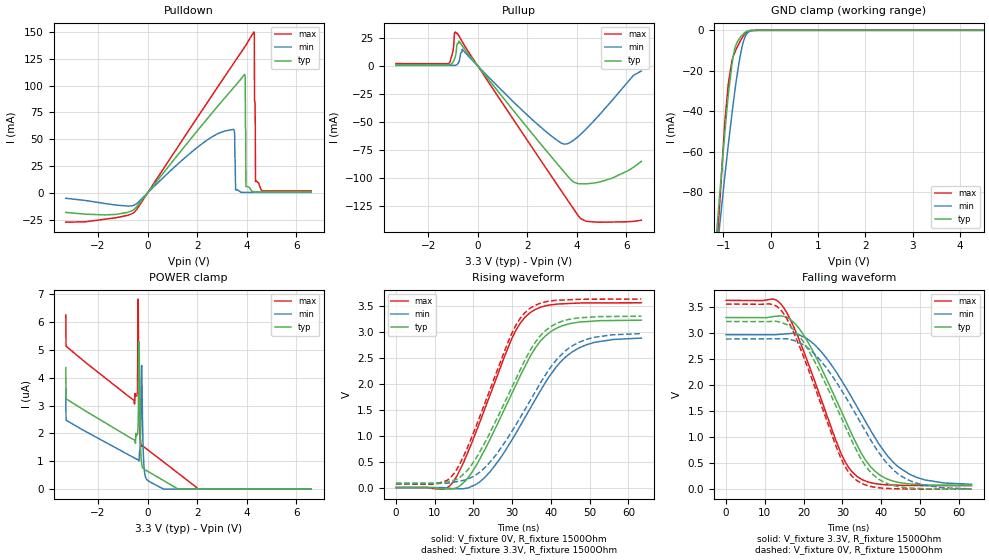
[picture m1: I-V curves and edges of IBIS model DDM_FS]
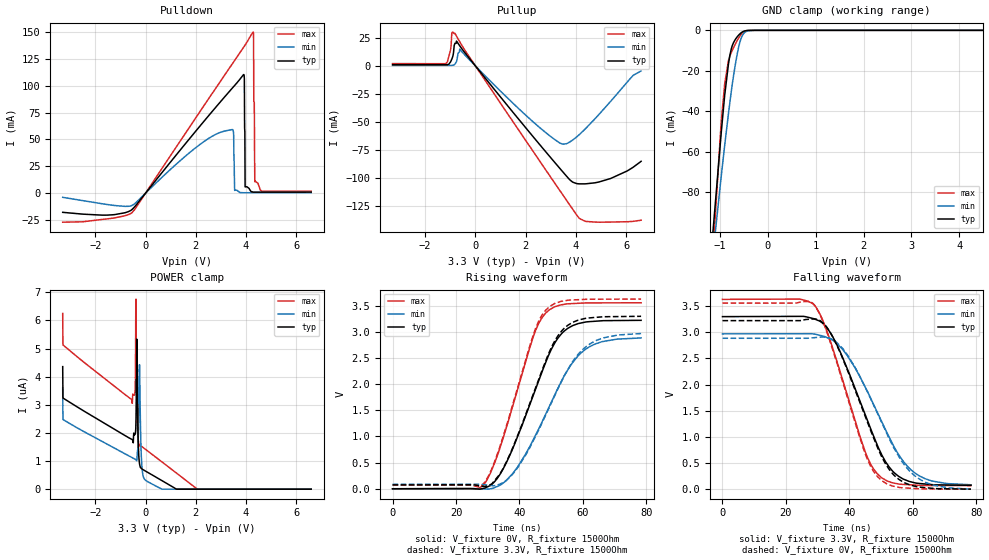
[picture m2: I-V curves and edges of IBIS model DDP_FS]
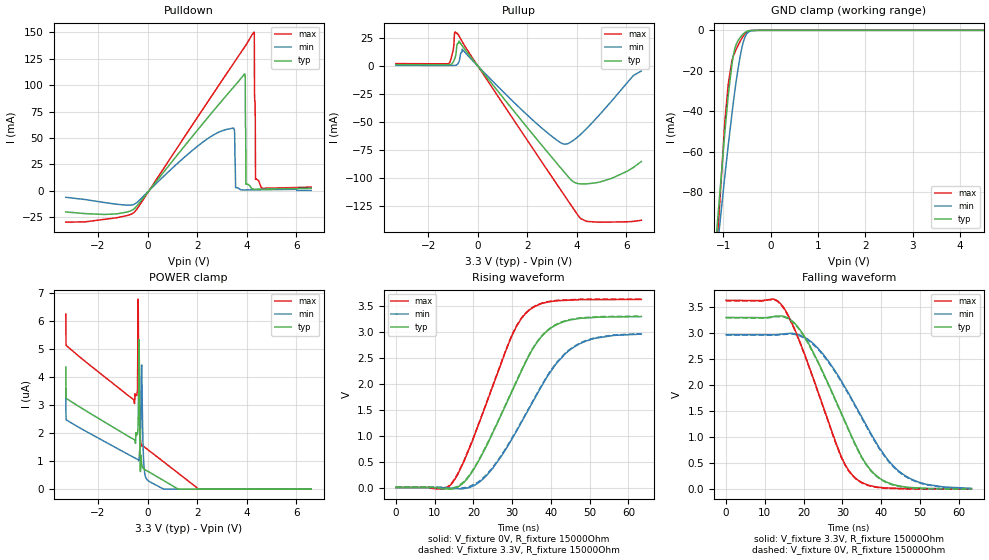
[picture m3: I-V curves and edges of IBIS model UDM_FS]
|Texas Instruments Incorporated
| ISOUSB111 Full/Low Speed Isolated USB Repeater
| Marketing Part # : ISOUSB111
| Package-type: SOIC
| #pins/pkg drawing : 16-pin DW
[IBIS Ver] 4.1
[File name] isousb211.ibs
[File Rev] 1.0
[Date] 09/25/2022
[Source]
| Texas Instruments Incorporated.
| 12500 TI Blvd
| Dallas, TX -75243
[Notes] Revision History:
| Rev 1.0: 09/25/2022
| - Initial version of the model
| - Model generated from simulations in TISPICE/SPECTRE
| - C_comp although listed in numerical order of value are
| obtained from varying PVT conditions. For PVT conditions for
| each specific value refer the buffer description under
| respective [Model]. IBIS model user is responsible for using
| appropriate C_comp to simulate for Signal Integrity.
| - Warnings regarding combined Non-monotonicity of various models have been
| reviewed and considered minor and can be ignored.
[Disclaimer]
| This model is designed as an aid for customers of Texas Instruments.
| TI and its licensors and suppliers make no warranties, either expressed
| or implied, with respect to this model, including the warranties of
| merchantability or fitness for a particular purpose. The model is
| provided solely on an "as is" basis. The entire risk as to its quality
| and performance is with the customer.
| This model is subject to change without notice. Texas Instruments
| Incorporated is not responsible for updating this model.
[Copyright]
(C) Copyright 2022 Texas Instruments Incorporated. All rights reserved.
[Component] ISOUSB211
[Manufacturer] Texas Instruments Incorporated
[Package]
R_pkg 0.05 0.04 0.06
L_pkg 1.5nH 1.2nH 2nH
C_pkg 0.2pF 0.16pF 0.24pF
| pin number (pin name) mapping to model name
[Pin] signal_name  model_name   R_pin   L_pin   C_pin
1 Vbus1 Power 0 0 0
2 V3p3V1 Power 0 0 0
3 GND1 GND 0 0 0
4 V1p8V1 Power 0 0 0
5 Vcc1 Power 0 0 0
6 V2OK NC 0 0 0
7 UDM UDM 0 0 0
8 UDP UDP 0 0 0
9 EQ10 NC 0 0 0
10 EQ11 NC 0 0 0
11 V1p8V1_2 Power 0 0 0
12 GND1 GND 0 0 0
13 CDPENZ1 NC 0 0 0
14 SDA1 NC 0 0 0
15 SDA2 NC 0 0 0
16 CDPENZ2 NC 0 0 0
17 GND2 GND 0 0 0
18 V1p8V2_2 Power 0 0 0
19 EQ21 NC 0 0 0
20 EQ20 NC 0 0 0
21 DDP DDP 0 0 0
22 DDM DDM 0 0 0
23 V1OK NC 0 0 0
24 Vcc2 Power 0 0 0
25 V1p8V2 Power 0 0 0
26 GND2 GND 0 0 0
27 V3p3V2 Power 0 0 0
28 Vbus2 Power 0 0 0
[Model Selector]   UDP
UDP_FS   upstream_positive_full_speed_mode
UDP_LS   upstream_positive_low_speed_mode
DP_EQ0   high_speed_eq0
DP_EQ1   high_speed_eq1
DP_EQ2   high_speed_eq2
DP_EQ3   high_speed_eq3
DP_EQ4   high_speed_eq4
DP_EQ5   high_speed_eq5
DP_EQ6   high_speed_eq6
DP_EQ7   high_speed_eq7
[Model Selector]   UDM
UDM_FS   upstream_negative_full_speed_mode
UDM_LS   upstream_negative_low_speed_mode
DM_EQ0   high_speed_eq0
DM_EQ1   high_speed_eq1
DM_EQ2   high_speed_eq2
DM_EQ3   high_speed_eq3
DM_EQ4   high_speed_eq4
DM_EQ5   high_speed_eq5
DM_EQ6   high_speed_eq6
DM_EQ7   high_speed_eq7
[Model Selector]   DDP
DDP_FS   downstream_positive_full_speed_mode
DDP_LS   downstream_positive_low_speed_mode
DP_EQ0   high_speed_eq0
DP_EQ1   high_speed_eq1
DP_EQ2   high_speed_eq2
DP_EQ3   high_speed_eq3
DP_EQ4   high_speed_eq4
DP_EQ5   high_speed_eq5
DP_EQ6   high_speed_eq6
DP_EQ7   high_speed_eq7
[Model Selector]   DDM
DDM_FS   downstream_negative_full_speed_mode
DDM_LS   downstream_negative_low_speed_mode
DM_EQ0   high_speed_eq0
DM_EQ1   high_speed_eq1
DM_EQ2   high_speed_eq2
DM_EQ3   high_speed_eq3
DM_EQ4   high_speed_eq4
DM_EQ5   high_speed_eq5
DM_EQ6   high_speed_eq6
DM_EQ7   high_speed_eq7
| Models and submodels in the file (24): UDP_LS (I/O), DDM_FS (I/O), DDM_LS (I/O), DDP_FS (I/O), DDP_LS (I/O), UDM_FS (I/O), UDM_LS (I/O), UDP_FS (I/O), DM_EQ0 (Output), DM_EQ1 (Output), DM_EQ2 (Output), DM_EQ3 (Output), DM_EQ4 (Output), DM_EQ5 (Output), DM_EQ6 (Output), DM_EQ7 (Output), DP_EQ0 (Output), DP_EQ1 (Output), DP_EQ2 (Output), DP_EQ3 (Output), DP_EQ4 (Output), DP_EQ5 (Output), DP_EQ6 (Output), DP_EQ7 (Output)
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[Model]   DDM_FS
Model_type   I/O
Polarity   Non-Inverting
Enable   Active-Low
Vinl = 0.8
Vinh = 2
Vmeas = 1.65
Vref = 1.65
Cref = 7pF
Rref = 15000
|   typ   min   max
C_comp   8pF   5pF   10pF
[Voltage Range]   3.3   2.97   3.63
[Temperature Range]   27   150   -40
[Pullup Reference]   3.3   2.97   3.63
[Pulldown Reference]   0   0   -0
[Power Clamp Reference]   3.3   2.97   3.63
[GND Clamp Reference]   0   0   0
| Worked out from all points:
|   slope of the pulldown table from 0 to 0.495 V, typ, clamps not added: 34.2 ohm
|   slope of the pullup table from 0 to 0.495 V, typ, clamps not added: 35.8 ohm
|   GND clamp passes 1 mA (typ) near -0.54 V on its own axis
|   falling waveform, V_fixture 3.3V, R_fixture 1500Ohm: 20-80 % time 12.3ns typ, 14.3ns min, 10.5ns max; typ from 3.3 V to 0.074 V
|   rising waveform, V_fixture 0V, R_fixture 1500Ohm: 20-80 % time 12.7ns typ, 14.1ns min, 11.1ns max; typ from 0 V to 3.22 V
|   rising waveform, V_fixture 3.3V, R_fixture 1500Ohm: 20-80 % time 12.9ns typ, 14.5ns min, 11.1ns max; typ from 0.073 V to 3.3 V
|   falling waveform, V_fixture 0V, R_fixture 1500Ohm: 20-80 % time 12.4ns typ, 14.5ns min, 10.6ns max; typ from 3.22 V to 0 V
[Pulldown]
|   Voltage   I(typ)   I(min)   I(max)
-3.3V     -18.2mA    -5.025mA   -27.3mA
-537.9mV  -15.2mA    -11.4mA    -18.05mA
3.452V    97.57mA    59.15mA    120.1mA
3.551V    100.2mA    2.565mA    123.5mA
3.917V    110.3mA    416.6uA    136mA
3.937V    106.9mA    416.6uA    136.7mA
3.967V    5.849mA    416.6uA    137.7mA
4.283V    1.079mA    416.7uA    149.8mA
4.303V    992.1uA    416.7uA    149.2mA
4.313V    991.4uA    416.7uA    86.59mA
4.353V    991.8uA    416.8uA    10.6mA
6.6V      1.045mA    452.9uA    1.865mA
[GND Clamp]
|   Voltage   I(typ)   I(min)   I(max)
-3.3V     -1.286A    -1.12A     -1.579A
-1.3V     -145.3mA   -147.2mA   -170.6mA
-973.5mV  -52.59mA   -73.66mA   -47.69mA
-894.3mV  -32.06mA   -56.82mA   -26.49mA
-815.1mV  -16.5mA    -41.06mA   -14.88mA
-785.4mV  -12.23mA   -35.46mA   -12.65mA
-735.9mV  -7.575mA   -26.62mA   -9.854mA
-627mV    -3.033mA   -10.97mA   -4.745mA
-567.6mV  -1.539mA   -5.066mA   -2.489mA
-498.3mV  -471.8uA   -1.572mA   -746.7uA
-260.7mV  0A         -5.306uA   0A
6.6V      0A         0A         0A
[Pullup]
|   Voltage   I(typ)   I(min)   I(max)
-3.3V     1.143mA    463.1uA    2.098mA
-1.181V   1.062mA    442.4uA    1.969mA
-993.3mV  3.464mA    442uA      14.04mA
-933.9mV  6.443mA    534.3uA    29.81mA
-815.1mV  20.24mA    1.625mA    29.16mA
-627mV    18.1mA     15mA       21.74mA
1.957V    -54.06mA   -43.1mA    -65.17mA
3.491V    -95.06mA   -70.03mA   -115.7mA
3.868V    -103.9mA   -66.45mA   -128mA
4.382V    -105.5mA   -56.25mA   -139.1mA
5.402V    -100.6mA   -31.33mA   -139.7mA
6.6V      -85.42mA   -4.486mA   -138.1mA
[POWER Clamp]
|   Voltage   I(typ)   I(min)   I(max)
-3.3V     4.356uA    3.599uA    6.245uA
-3.29V    3.24uA     2.477uA    5.129uA
-528mV    1.759uA    1.119uA    3.056uA
-409.2mV  1.967uA    1.064uA    3.479uA
-379.5mV  2.466uA    1.044uA    6.817uA
-349.8mV  5.299uA    1.01uA     3.356uA
-290.4mV  1.653uA    1.775uA    1.768uA
-250.8mV  990.4nA    4.213uA    1.556uA
-171.6mV  742.1nA    1.255uA    1.531uA
-62.7mV   674.2nA    386.2nA    1.457uA
2.056V    0A         0A         4.44nA
6.6V      0A         0A         0A
[Ramp]
R_load = 1500
|   typ   min   max
dV/dt_r   1.93262/1.26758e-08   1.7258/1.41041e-08   2.1342/1.10067e-08
dV/dt_f   1.93485/1.22744e-08   1.7255/1.42298e-08   2.13627/1.05125e-08
[Falling Waveform]
V_fixture = 3.3V
V_fixture_min = 2.97V
V_fixture_max = 3.63V
R_fixture = 1500Ohm
C_fixture = 0F
|   Time   V(typ)   V(min)   V(max)
0s        3.298V     2.969V     3.628V
14.55ns   3.324V     2.979V     3.522V
17.92ns   3.171V     2.984V     3.041V
22.88ns   2.584V     2.773V     2.078V
29.72ns   1.502V     2.098V     678.8mV
33.83ns   844.9mV    1.58V      243.3mV
38.29ns   354.9mV    1.008V     109.5mV
44.81ns   126.3mV    407.8mV    74.94mV
51.52ns   83.59mV    174.8mV    69.48mV
63.33ns   73.73mV    92.92mV    67.43mV
[Rising Waveform]
V_fixture = 0V
V_fixture_min = 0V
V_fixture_max = 0V
R_fixture = 1500Ohm
C_fixture = 0F
|   Time   V(typ)   V(min)   V(max)
0s        7.21nV     276nV      6.379nV
12.02ns   -25.13mV   -1.021mV   -31.53mV
14.55ns   -28.04mV   -21.32mV   87.57mV
17.92ns   127.4mV    -16.65mV   565.1mV
22.88ns   720.2mV    189.9mV    1.502V
30.16ns   1.847V     944.2mV    2.908V
34.59ns   2.517V     1.515V     3.364V
40.02ns   3.004V     2.182V     3.516V
45.64ns   3.165V     2.617V     3.546V
63.33ns   3.221V     2.876V     3.557V
[Rising Waveform]
V_fixture = 3.3V
V_fixture_min = 2.97V
V_fixture_max = 3.63V
R_fixture = 1500Ohm
C_fixture = 0F
|   Time   V(typ)   V(min)   V(max)
0s        73.38mV    83.93mV    67.42mV
10.05ns   74.06mV    82.64mV    70.96mV
15.13ns   142mV      106mV      283.6mV
18.84ns   367mV      174.1mV    839.2mV
24.36ns   1.069V     494.6mV    1.901V
30.07ns   1.952V     1.101V     2.994V
34.4ns    2.607V     1.643V     3.439V
39.75ns   3.089V     2.299V     3.589V
45.64ns   3.249V     2.733V     3.618V
63.33ns   3.298V     2.963V     3.628V
[Falling Waveform]
|Gnd
V_fixture = 0V
V_fixture_min = 0V
V_fixture_max = 0V
R_fixture = 1500Ohm
C_fixture = 0F
|   Time   V(typ)   V(min)   V(max)
0s        3.222V     2.885V     3.557V
11.28ns   3.221V     2.889V     3.561V
14.55ns   3.195V     2.89V      3.404V
18.84ns   2.946V     2.817V     2.761V
22.88ns   2.449V     2.595V     1.969V
29.64ns   1.389V     1.918V     592.2mV
33.63ns   753.5mV    1.42V      172.6mV
39.25ns   198.2mV    720mV      28.06mV
45.64ns   36.48mV    232.3mV    4.575mV
63.33ns   223.6uV    5.519mV    8.818uV
[Model]   DDP_FS
Model_type   I/O
Polarity   Non-Inverting
Enable   Active-Low
Vinl = 0.8
Vinh = 2
Vmeas = 1.65
Vref = 1.65
Cref = 7pF
Rref = 15000
|   typ   min   max
C_comp   8pF   5pF   10pF
[Voltage Range]   3.3   2.97   3.63
[Temperature Range]   27   150   -40
[Pullup Reference]   3.3   2.97   3.63
[Pulldown Reference]   -0   0   0
[Power Clamp Reference]   3.3   2.97   3.63
[GND Clamp Reference]   0   0   0
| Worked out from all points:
|   slope of the pulldown table from 0 to 0.495 V, typ, clamps not added: 34.2 ohm
|   slope of the pullup table from 0 to 0.495 V, typ, clamps not added: 35.8 ohm
|   GND clamp passes 1 mA (typ) near -0.54 V on its own axis
|   falling waveform, V_fixture 3.3V, R_fixture 1500Ohm: 20-80 % time 12.8ns typ, 14.5ns min, 11.1ns max; typ from 3.3 V to 0.073 V
|   rising waveform, V_fixture 0V, R_fixture 1500Ohm: 20-80 % time 12.4ns typ, 14.5ns min, 10.6ns max; typ from 0 V to 3.22 V
|   rising waveform, V_fixture 3.3V, R_fixture 1500Ohm: 20-80 % time 12.3ns typ, 14.2ns min, 10.5ns max; typ from 0.073 V to 3.3 V
|   falling waveform, V_fixture 0V, R_fixture 1500Ohm: 20-80 % time 12.7ns typ, 14.1ns min, 11ns max; typ from 3.22 V to 0 V
[Pulldown]
|   Voltage   I(typ)   I(min)   I(max)
-3.3V     -17.81mA   -3.85mA    -26.98mA
-537.9mV  -15.2mA    -11.4mA    -18.05mA
3.452V    97.57mA    59.13mA    120.1mA
3.551V    100.2mA    2.568mA    123.5mA
3.907V    110.2mA    416.5uA    135.6mA
3.937V    106.3mA    416.5uA    136.7mA
3.967V    5.859mA    416.5uA    137.7mA
4.283V    1.074mA    416.6uA    149.8mA
4.303V    991.3uA    416.6uA    149mA
4.313V    991.1uA    416.6uA    85.12mA
4.353V    991.5uA    416.7uA    10.62mA
6.6V      1.044mA    452.8uA    1.864mA
[GND Clamp]
|   Voltage   I(typ)   I(min)   I(max)
-3.3V     -1.286A    -1.121A    -1.579A
-1.3V     -145.3mA   -147.2mA   -170.6mA
-973.5mV  -52.59mA   -73.66mA   -47.68mA
-894.3mV  -32.06mA   -56.81mA   -26.49mA
-815.1mV  -16.5mA    -41.06mA   -14.88mA
-785.4mV  -12.23mA   -35.46mA   -12.65mA
-735.9mV  -7.575mA   -26.62mA   -9.853mA
-627mV    -3.033mA   -10.97mA   -4.745mA
-567.6mV  -1.539mA   -5.066mA   -2.489mA
-498.3mV  -471.8uA   -1.571mA   -746.6uA
-260.7mV  0A         -5.306uA   0A
6.6V      0A         0A         0A
[Pullup]
|   Voltage   I(typ)   I(min)   I(max)
-3.3V     1.143mA    463.2uA    2.099mA
-1.181V   1.062mA    442.5uA    1.996mA
-993.3mV  3.496mA    442.2uA    14.19mA
-933.9mV  6.482mA    535.1uA    29.92mA
-815.1mV  20.26mA    1.636mA    29.12mA
-627mV    18.09mA    14.99mA    21.7mA
1.957V    -54.04mA   -43.09mA   -65.14mA
3.491V    -95.04mA   -70.01mA   -115.7mA
3.868V    -103.9mA   -66.43mA   -128mA
4.382V    -105.5mA   -56.22mA   -139.1mA
5.392V    -100.7mA   -31.56mA   -139.7mA
6.6V      -85.38mA   -4.479mA   -138.1mA
[POWER Clamp]
|   Voltage   I(typ)   I(min)   I(max)
-3.3V     4.356uA    3.599uA    6.245uA
-3.29V    3.24uA     2.478uA    5.13uA
-528mV    1.759uA    1.119uA    3.053uA
-409.2mV  1.963uA    1.064uA    3.57uA
-379.5mV  2.509uA    1.044uA    6.758uA
-349.8mV  5.335uA    1.011uA    3.278uA
-300.3mV  1.978uA    1.538uA    1.841uA
-250.8mV  984.9nA    4.227uA    1.559uA
-171.6mV  741.8nA    1.249uA    1.531uA
-62.7mV   674.2nA    385.9nA    1.457uA
2.056V    0A         0A         4.445nA
6.6V      0A         0A         0A
[Ramp]
R_load = 1500
|   typ   min   max
dV/dt_r   1.93339/1.2374e-08   1.73122/1.44206e-08   2.13488/1.05473e-08
dV/dt_f   1.93542/1.282e-08   1.73113/1.44351e-08   2.13691/1.10541e-08
[Falling Waveform]
V_fixture = 3.3V
V_fixture_min = 2.97V
V_fixture_max = 3.63V
R_fixture = 1500Ohm
C_fixture = 0F
|   Time   V(typ)   V(min)   V(max)
0s        3.299V     2.969V     3.629V
28.18ns   3.269V     2.972V     3.559V
31.52ns   3.176V     2.93V      3.243V
35.96ns   2.774V     2.79V      2.466V
44.98ns   1.428V     1.953V     717.8mV
48.64ns   866.3mV    1.491V     304.5mV
53.85ns   331.6mV    836.3mV    118.6mV
60.64ns   121mV      310mV      78.34mV
66.13ns   86.39mV    154.8mV    70.52mV
78.33ns   73.35mV    83.9mV     67.4mV
[Rising Waveform]
V_fixture = 0V
V_fixture_min = 0V
V_fixture_max = 0V
R_fixture = 1500Ohm
C_fixture = 0F
|   Time   V(typ)   V(min)   V(max)
0s        -34.15uV   -42.85uV   -28.52uV
28.18ns   733.5uV    -529.6uV   47.19mV
30.77ns   61.93mV    -1.109mV   288.8mV
35.96ns   510.8mV    166.9mV    1.189V
44.25ns   1.771V     927.5mV    2.891V
47.96ns   2.37V      1.388V     3.341V
53.29ns   2.969V     2.065V     3.519V
60.64ns   3.187V     2.66V      3.555V
66.13ns   3.214V     2.815V     3.556V
78.33ns   3.222V     2.885V     3.558V
[Rising Waveform]
V_fixture = 3.3V
V_fixture_min = 2.97V
V_fixture_max = 3.63V
R_fixture = 1500Ohm
C_fixture = 0F
|   Time   V(typ)   V(min)   V(max)
0s        73.35mV    83.9mV     67.4mV
28.18ns   49.36mV    81.55mV    69.35mV
30.77ns   77.31mV    63.43mV    311.4mV
34.85ns   389.1mV    118.5mV    999.2mV
44.34ns   1.81V      918.4mV    2.944V
48.15ns   2.427V     1.396V     3.408V
53.29ns   3.018V     2.058V     3.586V
60.19ns   3.251V     2.678V     3.622V
66.52ns   3.291V     2.888V     3.627V
78.33ns   3.299V     2.969V     3.629V
[Falling Waveform]
|Gnd
V_fixture = 0V
V_fixture_min = 0V
V_fixture_max = 0V
R_fixture = 1500Ohm
C_fixture = 0F
|   Time   V(typ)   V(min)   V(max)
0s        3.222V     2.885V     3.558V
28.18ns   3.252V     2.893V     3.567V
32.92ns   3.095V     2.9V       3.001V
37.88ns   2.501V     2.691V     2.057V
44.72ns   1.437V     1.982V     722.9mV
48.74ns   817.9mV    1.466V     248.5mV
53.85ns   282mV      810.6mV    57.69mV
60.64ns   56.6mV     254.8mV    12.31mV
66.52ns   14.49mV    76.61mV    3.507mV
78.33ns   -34.15uV   -42.85uV   -28.52uV
[Model]   UDM_FS
Model_type   I/O
Polarity   Non-Inverting
Enable   Active-Low
Vinl = 0.8
Vinh = 2
Vmeas = 1.65
Vref = 1.65
Cref = 7pF
Rref = 15000
|   typ   min   max
C_comp   8pF   5pF   10pF
[Voltage Range]   3.3   2.97   3.63
[Temperature Range]   27   150   -40
[Pullup Reference]   3.3   2.97   3.63
[Pulldown Reference]   -0   -0   -0
[Power Clamp Reference]   3.3   2.97   3.63
[GND Clamp Reference]   0   0   0
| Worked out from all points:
|   slope of the pulldown table from 0 to 0.495 V, typ, clamps not added: 33.7 ohm
|   slope of the pullup table from 0 to 0.495 V, typ, clamps not added: 35.8 ohm
|   GND clamp passes 1 mA (typ) near -0.54 V on its own axis
|   falling waveform, V_fixture 3.3V, R_fixture 15000Ohm: 20-80 % time 12.3ns typ, 14.2ns min, 10.5ns max; typ from 3.3 V to 0.008 V
|   rising waveform, V_fixture 0V, R_fixture 15000Ohm: 20-80 % time 12.6ns typ, 14.1ns min, 11ns max; typ from 0 V to 3.29 V
|   rising waveform, V_fixture 3.3V, R_fixture 15000Ohm: 20-80 % time 12.7ns typ, 14.1ns min, 11ns max; typ from 0.007 V to 3.3 V
|   falling waveform, V_fixture 0V, R_fixture 15000Ohm: 20-80 % time 12.3ns typ, 14.2ns min, 10.5ns max; typ from 3.29 V to 0 V
[Pulldown]
|   Voltage   I(typ)   I(min)   I(max)
-3.3V     -19.93mA   -6.107mA   -29.66mA
-537.9mV  -16.94mA   -12.7mA    -20.3mA
3.452V    97.68mA    59.35mA    120.1mA
3.551V    100.4mA    2.79mA     123.5mA
3.917V    110.6mA    791.1uA    136.2mA
3.937V    107.5mA    798uA      136.9mA
3.967V    6.141mA    808.4uA    138mA
4.283V    1.56mA     916.9uA    150.2mA
4.303V    1.492mA    923.6uA    149.6mA
4.343V    1.509mA    936.8uA    69.22mA
4.353V    1.513mA    940.1uA    10.96mA
6.6V      2.508mA    452.9uA    3.524mA
[GND Clamp]
|   Voltage   I(typ)   I(min)   I(max)
-3.3V     -1.286A    -1.12A     -1.579A
-1.3V     -145.3mA   -147.2mA   -170.6mA
-973.5mV  -52.59mA   -73.66mA   -47.69mA
-894.3mV  -32.06mA   -56.82mA   -26.49mA
-815.1mV  -16.5mA    -41.06mA   -14.88mA
-785.4mV  -12.23mA   -35.46mA   -12.65mA
-735.9mV  -7.575mA   -26.62mA   -9.854mA
-627mV    -3.033mA   -10.97mA   -4.745mA
-567.6mV  -1.539mA   -5.066mA   -2.489mA
-498.3mV  -471.8uA   -1.572mA   -746.7uA
-260.7mV  0A         -5.306uA   0A
6.6V      0A         0A         0A
[Pullup]
|   Voltage   I(typ)   I(min)   I(max)
-3.3V     1.142mA    462.6uA    2.095mA
-1.181V   1.061mA    442uA      1.922mA
-993.3mV  3.358mA    441.5uA    13.7mA
-933.9mV  6.314mA    531.1uA    29.51mA
-815.1mV  20.17mA    1.584mA    29.25mA
-627mV    18.16mA    15.03mA    21.83mA
1.957V    -54.04mA   -43.08mA   -65.14mA
3.501V    -95.32mA   -70.05mA   -116.1mA
3.868V    -103.9mA   -66.47mA   -128mA
4.392V    -105.6mA   -56.06mA   -139.2mA
5.412V    -100.6mA   -31.15mA   -139.8mA
6.6V      -85.55mA   -4.486mA   -138.2mA
[POWER Clamp]
|   Voltage   I(typ)   I(min)   I(max)
-3.3V     4.356uA    3.599uA    6.245uA
-3.29V    3.24uA     2.477uA    5.129uA
-528mV    1.759uA    1.119uA    3.053uA
-409.2mV  1.977uA    1.064uA    3.528uA
-379.5mV  2.534uA    1.044uA    6.78uA
-349.8mV  5.335uA    1.011uA    3.323uA
-290.4mV  625.9nA    1.782uA    1.767uA
-250.8mV  987.2nA    4.223uA    1.563uA
-171.6mV  742.1nA    1.25uA     1.531uA
-82.5mV   684.7nA    428.7nA    1.471uA
2.056V    0A         0A         4.456nA
6.6V      0A         0A         0A
[Ramp]
R_load = 15000
|   typ   min   max
dV/dt_r   1.97313/1.26192e-08   1.77083/1.40324e-08   2.1712/1.09691e-08
dV/dt_f   1.97353/1.22096e-08   1.77092/1.41056e-08   2.17144/1.04715e-08
[Falling Waveform]
V_fixture = 3.3V
V_fixture_min = 2.97V
V_fixture_max = 3.63V
R_fixture = 15000Ohm
C_fixture = 0F
|   Time   V(typ)   V(min)   V(max)
0s        3.297V     2.968V     3.626V
12.09ns   3.313V     2.966V     3.651V
14.66ns   3.322V     2.98V      3.508V
18.36ns   3.132V     2.974V     2.956V
23.41ns   2.494V     2.732V     1.94V
29.8ns    1.452V     2.071V     611.3mV
33.82ns   791.7mV    1.546V     184.7mV
38.3ns    290.3mV    950.3mV    49.6mV
46.09ns   44.79mV    264.6mV    10.76mV
63.33ns   7.77mV     16.09mV    6.866mV
[Rising Waveform]
V_fixture = 0V
V_fixture_min = 0V
V_fixture_max = 0V
R_fixture = 15000Ohm
C_fixture = 0F
|   Time   V(typ)   V(min)   V(max)
0s        7.357nV    283.2nV    6.487nV
12.09ns   -26.05mV   -1.027mV   -31.65mV
14.66ns   -27.01mV   -14.92mV   98.06mV
18.36ns   166.2mV    -9.284mV   647.7mV
23.41ns   806mV      231.7mV    1.63V
30.23ns   1.895V     971.2mV    2.971V
34.59ns   2.572V     1.549V     3.424V
40.03ns   3.071V     2.241V     3.579V
45.63ns   3.232V     2.687V     3.608V
63.33ns   3.289V     2.951V     3.619V
[Rising Waveform]
V_fixture = 3.3V
V_fixture_min = 2.97V
V_fixture_max = 3.63V
R_fixture = 15000Ohm
C_fixture = 0F
|   Time   V(typ)   V(min)   V(max)
0s        7.485mV    8.596mV    6.856mV
12.09ns   -13.82mV   7.096mV    -17.8mV
14.66ns   -7.906mV   -9.264mV   111.8mV
18.36ns   181.9mV    8.119mV    659.8mV
23.41ns   819.4mV    250.8mV    1.641V
30.23ns   1.907V     987.8mV    2.981V
34.59ns   2.584V     1.566V     3.432V
40.03ns   3.081V     2.259V     3.587V
45.63ns   3.241V     2.699V     3.615V
63.33ns   3.296V     2.96V      3.626V
[Falling Waveform]
|Gnd
V_fixture = 0V
V_fixture_min = 0V
V_fixture_max = 0V
R_fixture = 15000Ohm
C_fixture = 0F
|   Time   V(typ)   V(min)   V(max)
0s        3.289V     2.959V     3.619V
12.09ns   3.304V     2.957V     3.64V
14.66ns   3.309V     2.969V     3.497V
18.36ns   3.117V     2.962V     2.945V
23.41ns   2.481V     2.713V     1.929V
29.73ns   1.451V     2.058V     613.7mV
33.77ns   788mV      1.534V     179.6mV
38.3ns    279.9mV    931.6mV    40.96mV
46.09ns   36.64mV    251.2mV    3.861mV
63.33ns   271.3uV    7.115mV    10.05uV
